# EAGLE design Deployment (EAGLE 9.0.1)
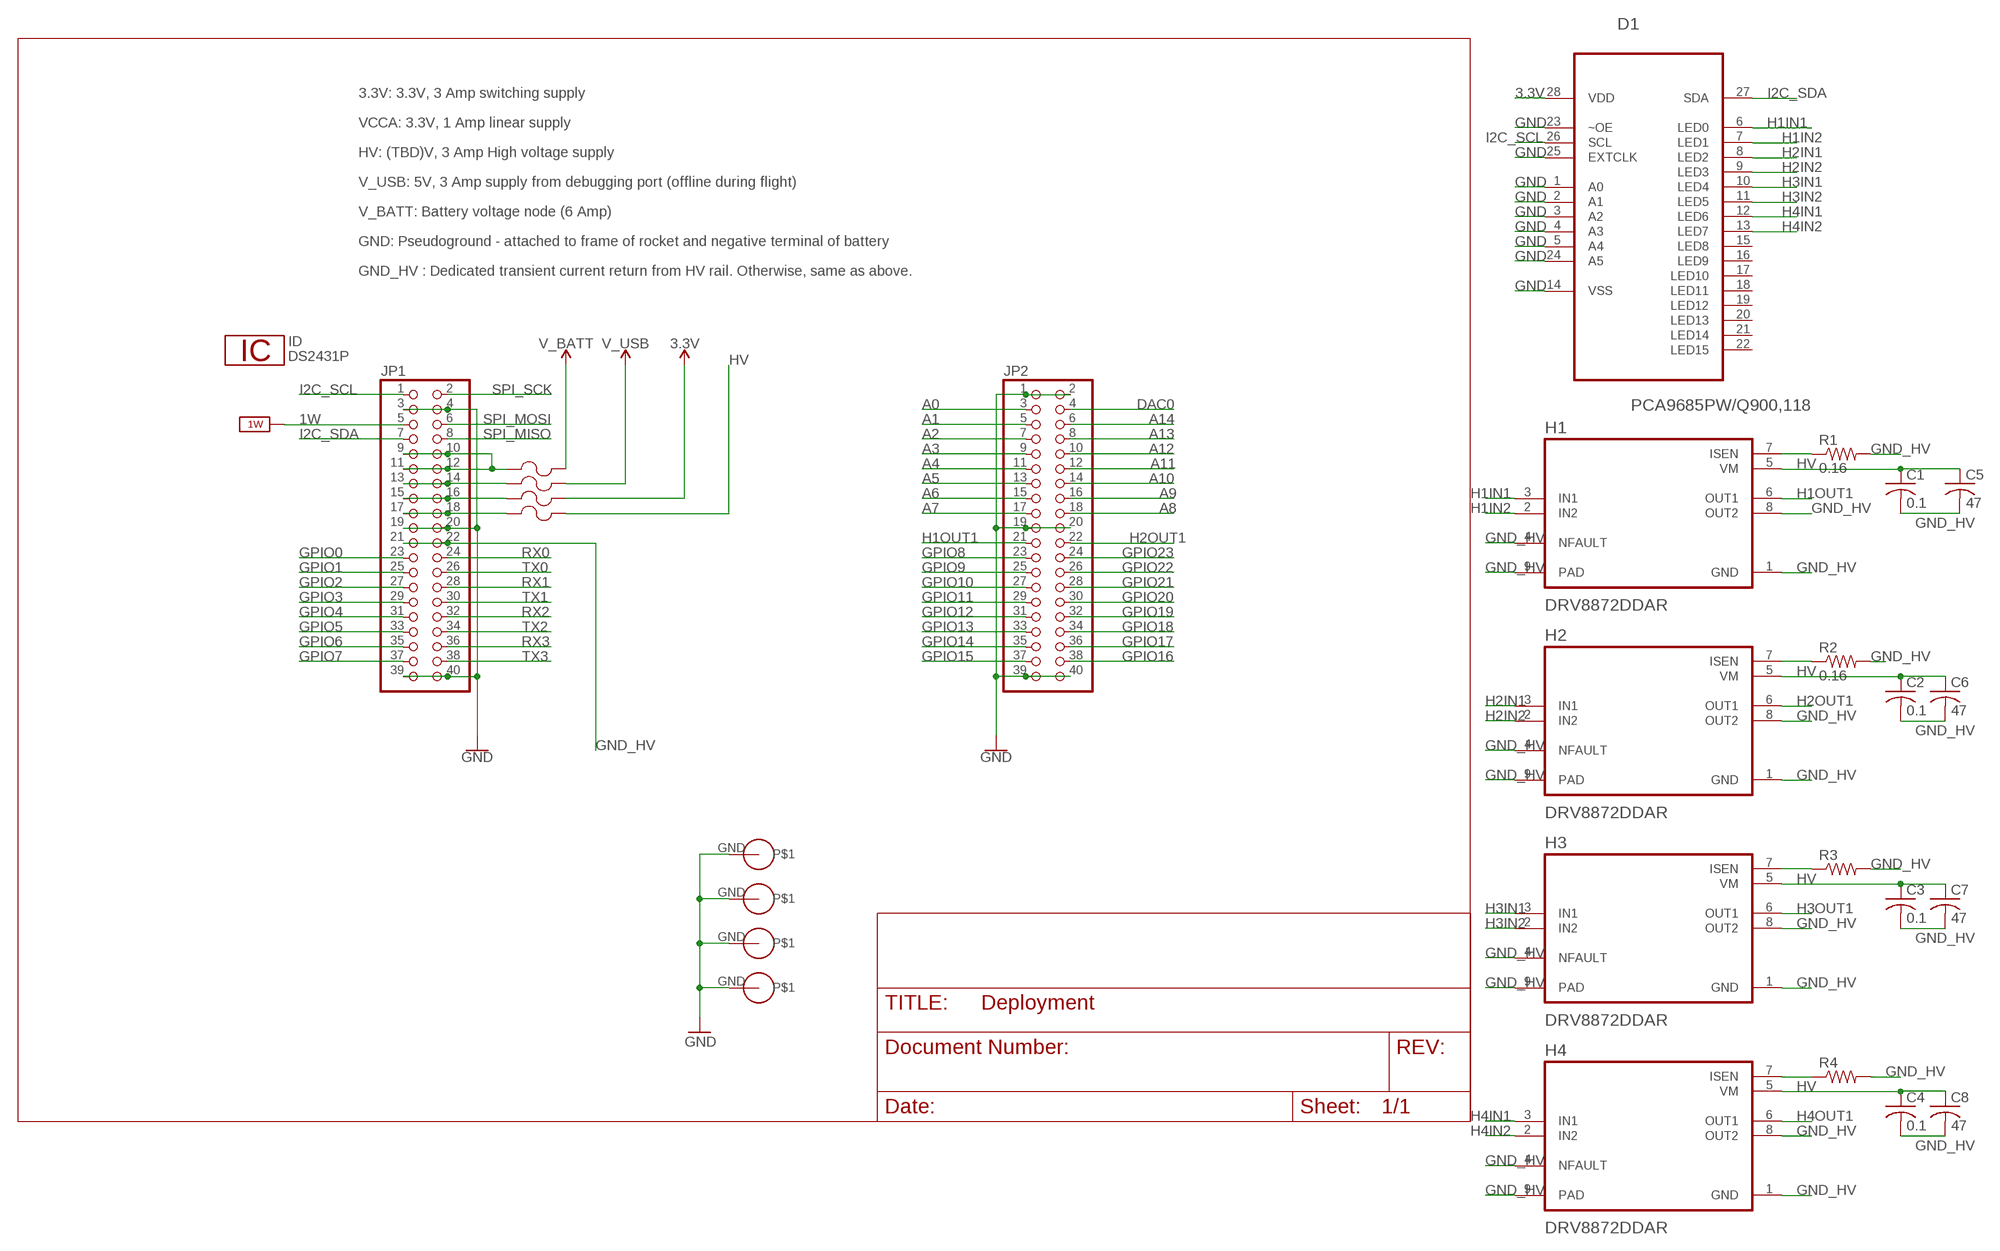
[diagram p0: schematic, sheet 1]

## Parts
C1  0.1  C-USC0805  [C0805]
C2  0.1  C-USC0805  [C0805]
C3  0.1  C-USC0805  [C0805]
C4  0.1  C-USC0805  [C0805]
C5  47  C-USC0805  [C0805]
C6  47  C-USC0805  [C0805]
C7  47  C-USC0805  [C0805]
C8  47  C-USC0805  [C0805]
D1  PCA9685PW/Q900,118  [SOP65P640X110-28N]
F1  0603SFF150F/32-2  [FUS0603_TYCO]
F2  0603SFF150F/32-2  [FUS0603_TYCO]
F3  0603SFF150F/32-2  [FUS0603_TYCO]
F4  0603SFF150F/32-2  [FUS0603_TYCO]
H1  DRV8872DDAR  [SOIC127P600X170-8N]
H2  DRV8872DDAR  [SOIC127P600X170-8N]
H3  DRV8872DDAR  [SOIC127P600X170-8N]
H4  DRV8872DDAR  [SOIC127P600X170-8N]
ID  DS2431P  [TSOC6]
JP1  PINHD-2X20  [2X20]
JP2  PINHD-2X20  [2X20]
R1  0.16  R-US_R1206  [R1206]
R2  0.16  R-US_R1206  [R1206]
R3  R-US_R1206  [R1206]
R4  R-US_R1206  [R1206]
U$1  PS/104-MOUNTING-HOLE  [PC/104-MOUNTING-HOLE]
U$2  PS/104-MOUNTING-HOLE  [PC/104-MOUNTING-HOLE]
U$3  PS/104-MOUNTING-HOLE  [PC/104-MOUNTING-HOLE]
U$4  PS/104-MOUNTING-HOLE  [PC/104-MOUNTING-HOLE]

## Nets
1W: JP1.5 ; supply symbol labelled 1W_SUP
3.3V: D1.28(VDD) F3.2
A0: JP2.3
A1: JP2.5
A2: JP2.7
A3: JP2.9
A4: JP2.11
A5: JP2.13
A6: JP2.15
A7: JP2.17
A8: JP2.18
A9: JP2.16
A10: JP2.14
A11: JP2.12
A12: JP2.10
A13: JP2.8
A14: JP2.6
DAC0: JP2.4
GND: D1.1(A0) D1.2(A1) D1.3(A2) D1.4(A3) D1.5(A4) D1.14(VSS) D1.23(~OE) D1.24(A5) D1.25(EXTCLK) JP1.3 JP1.4 JP1.19 JP1.20 JP1.39 JP1.40 JP2.1 JP2.2 JP2.19 JP2.20 JP2.39 JP2.40 U$1.GND U$2.GND U$3.GND U$4.GND
GND_HV: C1.2 C2.2 C3.2 C4.2 C5.2 C6.2 C7.2 C8.2 H1.1(GND) H1.4(NFAULT) H1.8(OUT2) H1.9(PAD) H2.1(GND) H2.4(NFAULT) H2.8(OUT2) H2.9(PAD) H3.1(GND) H3.4(NFAULT) H3.8(OUT2) H3.9(PAD) H4.1(GND) H4.4(NFAULT) H4.8(OUT2) H4.9(PAD) JP1.21 JP1.22 R1.2 R2.2 R3.2 R4.2
GPIO0: JP1.23
GPIO1: JP1.25
GPIO2: JP1.27
GPIO3: JP1.29
GPIO4: JP1.31
GPIO5: JP1.33
GPIO6: JP1.35
GPIO7: JP1.37
GPIO8: JP2.23
GPIO9: JP2.25
GPIO10: JP2.27
GPIO11: JP2.29
GPIO12: JP2.31
GPIO13: JP2.33
GPIO14: JP2.35
GPIO15: JP2.37
GPIO16: JP2.38
GPIO17: JP2.36
GPIO18: JP2.34
GPIO19: JP2.32
GPIO20: JP2.30
GPIO21: JP2.28
GPIO22: JP2.26
GPIO23: JP2.24
H1IN1: D1.6(LED0) H1.3(IN1)
H1IN2: D1.7(LED1) H1.2(IN2)
H1OUT1: H1.6(OUT1) JP2.21
H2IN1: D1.8(LED2) H2.3(IN1)
H2IN2: D1.9(LED3) H2.2(IN2)
H2OUT1: H2.6(OUT1) JP2.22
H3IN1: D1.10(LED4) H3.3(IN1)
H3IN2: D1.11(LED5) H3.2(IN2)
H3OUT1: H3.6(OUT1)
H4IN1: D1.12(LED6) H4.3(IN1)
H4IN2: D1.13(LED7) H4.2(IN2)
H4OUT1: H4.6(OUT1)
HV: C1.1 C2.1 C3.1 C4.1 C5.1 C6.1 C7.1 C8.1 F4.2 H1.5(VM) H2.5(VM) H3.5(VM) H4.5(VM)
I2C_SCL: D1.26(SCL) JP1.1
I2C_SDA: D1.27(SDA) JP1.7
N$1: F4.1 JP1.17 JP1.18
N$2: F2.1 JP1.13 JP1.14
N$3: F3.1 JP1.15 JP1.16
N$4: F1.1 JP1.9 JP1.10 JP1.11 JP1.12
N$5: H1.7(ISEN) R1.1
N$6: H2.7(ISEN) R2.1
N$10: H3.7(ISEN) R3.1
N$11: H4.7(ISEN) R4.1
RX0: JP1.24
RX1: JP1.28
RX2: JP1.32
RX3: JP1.36
SPI_MISO: JP1.8
SPI_MOSI: JP1.6
SPI_SCK: JP1.2
TX0: JP1.26
TX1: JP1.30
TX2: JP1.34
TX3: JP1.38
V_BATT: F1.2
V_USB: F2.2
Unconnected: D1.15(LED8) D1.16(LED9) D1.17(LED10) D1.18(LED11) D1.19(LED12) D1.20(LED13) D1.21(LED14) D1.22(LED15)

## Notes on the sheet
- 3.3V: 3.3V, 3 Amp switching supply
- VCCA: 3.3V, 1 Amp linear supply
- HV: (TBD)V, 3 Amp High voltage supply
- V_USB: 5V, 3 Amp supply from debugging port (offline during flight)
- V_BATT: Battery voltage node (6 Amp)
- GND: Pseudoground - attached to frame of rocket and negative terminal of battery
- GND_HV : Dedicated transient current return from HV rail. Otherwise, same as above.

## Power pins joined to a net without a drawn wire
1W: ID.2(1W)
GND: ID.1(GND)

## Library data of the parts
C1-C8 = resistor:C-US: CAPACITOR, American symbol
D1 = PCA9685PW_Q900_118:PCA9685PW/Q900,118: 16-channel, 12-bit PWM Fm+ I2C-bus LED controller; DESCRIPTION: PCA9685 Series 25 mA 5.5V 1 MHz 16-Ch 12-bit PWM Fm+ I2C-bus LED Controller; DIGI-KEY_PART_NUMBER: 568-5931-1-ND; DIGI-KEY_PURCHASE_URL: https://www.digikey.com/product-detail/en/nxp-usa-inc/PCA9685PW-Q900,118/568-5931-1-ND/2531218?utm_source=snapeda&utm_medium=aggregator&utm_campaign=symbol; MF: NXP USA; MP: PCA9685PW/Q900,118; PACKAGE: TSSOP-28 NXP Semiconductors
F1-F4 = CU inSpace 2019 Parts:0603SFF150F/32-2; MANUFACTURER_PART_NUMBER: 0603SFF150F322; VENDOR: Littelfuse Inc
H1-H4 = DRV8872DDAR:DRV8872DDAR: None; AVAILABILITY: Unavailable; DESCRIPTION: Brushed DC Motor Driver With PWM Control 6.5V to 45V 8-Pin SOPowerPAD T/R; MF: Texas Instruments; MP: DRV8872DDAR; PACKAGE: SO-8 Texas Instruments; PRICE: None
ID = 1wire:DS2431: 1024-Bit EEPROM
JP1 JP2 = pinhead:PINHD-2X20: PIN HEADER
R1-R4 = resistor:R-US_: RESISTOR, American symbol
U$1-U$4 = CU inSpace 2019 Parts:PS/104-MOUNTING-HOLE: Mounting hole for PC/104 board.

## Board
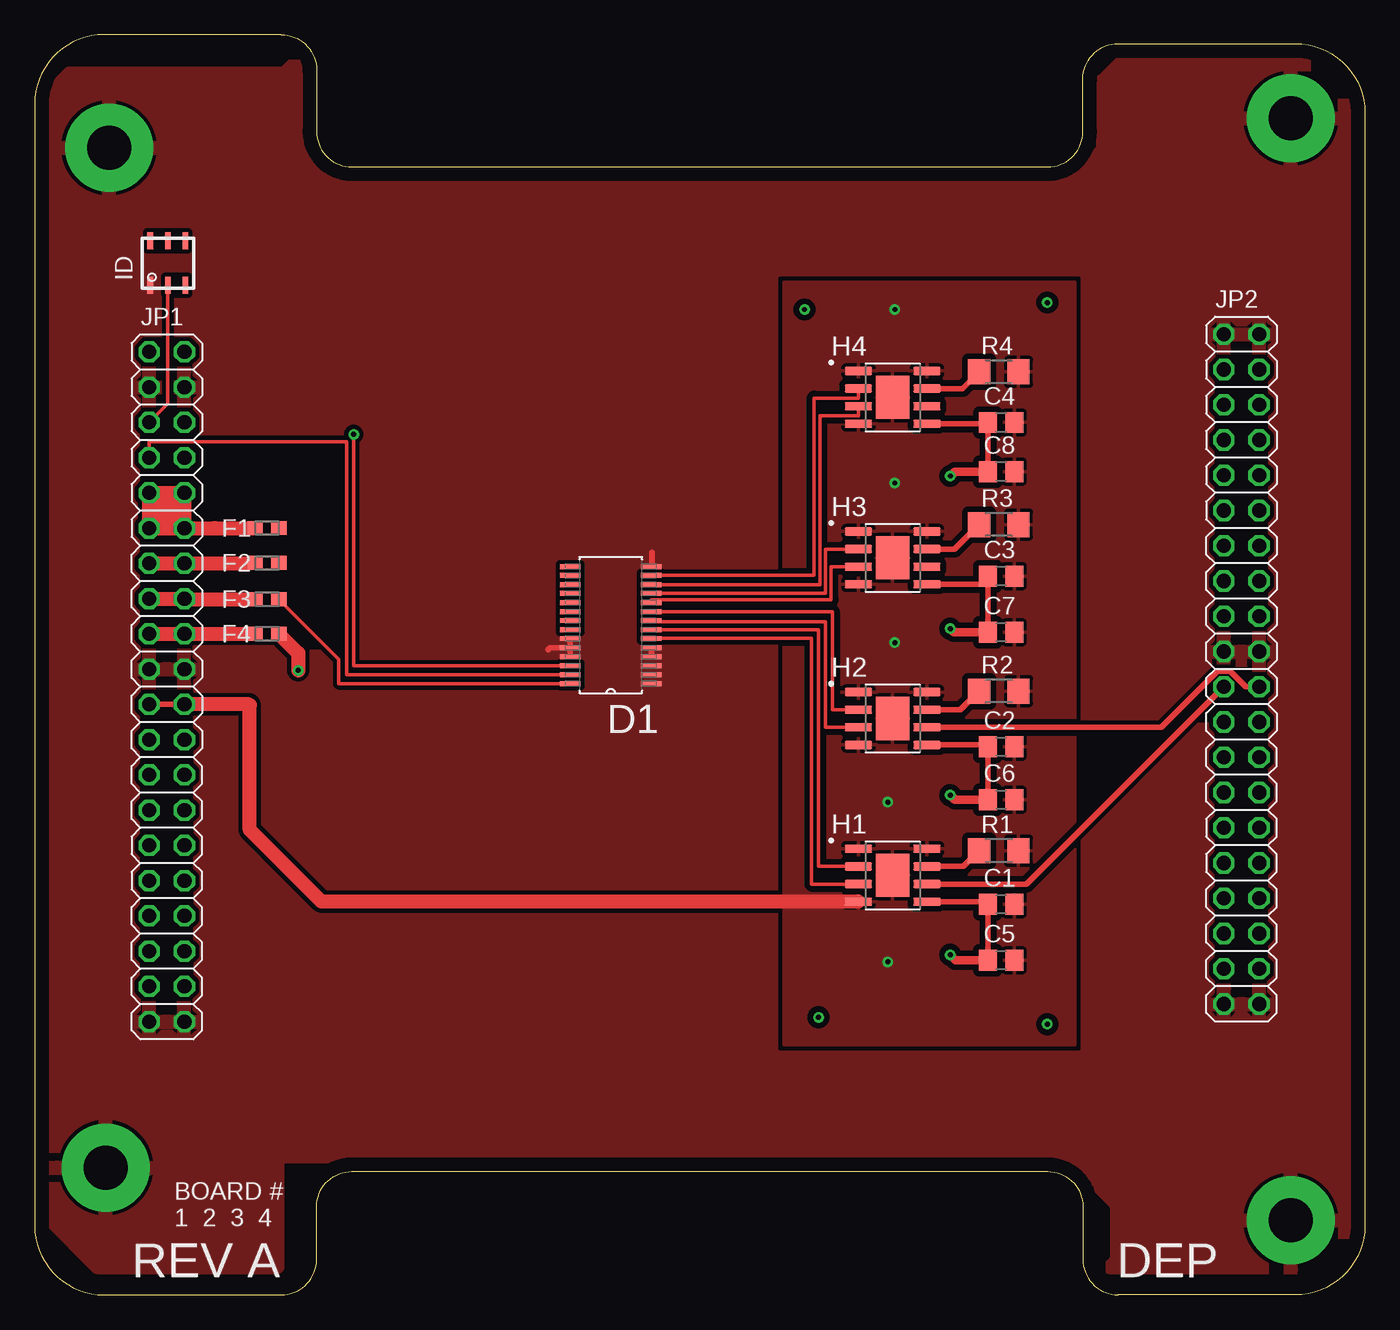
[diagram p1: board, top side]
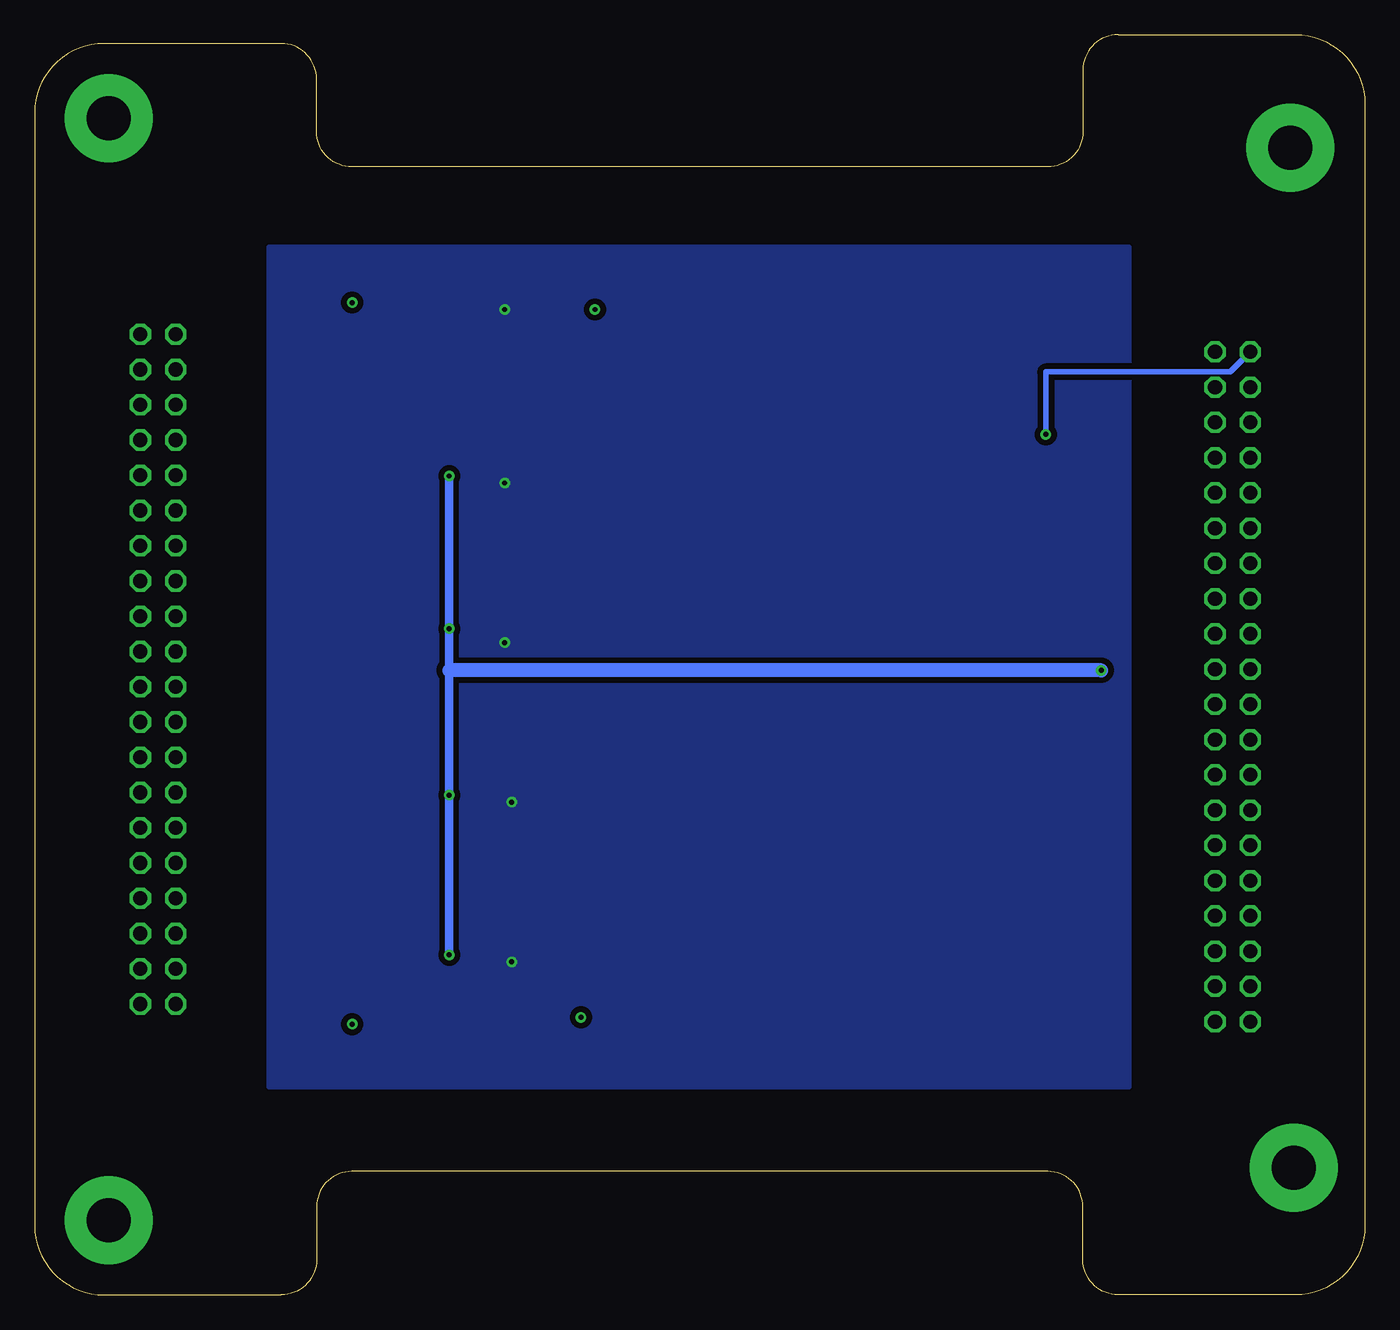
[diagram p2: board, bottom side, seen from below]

Size 95.89 x 90.81 mm. Coordinates in mm from the lower left corner, seen from the top.
Outline: 0,85.81 0,5 arc90 5,0 17.78,0 arc90 20.32,2.54 20.32,6.35 arc-90 22.86,8.89 73.03,8.89 arc-90 75.56,6.35 75.56,2.54 arc90 78.11,0 90.89,0 arc90 95.89,5 95.89,85.17 arc90 90.89,90.17 78.11,90.17 arc90 75.56,87.63 75.56,83.82 arc-90 73.03,81.28 22.86,81.28 arc-90 20.32,83.82 20.32,88.27 arc90 17.78,90.81 5,90.81 arc90 0,85.81
Copper layers (1*16): Top 0.035mm / dielectric 1.5mm / Bottom 0.035mm
Design rules "default": minimum track width 6mil, minimum drill 0.35mm, track to track 6mil, track to pad 6mil, pad to pad 6mil, via to via 6mil, smd to smd 6mil, copper to edge 40mil, drill to drill 6mil, minimum pad ring 10mil, minimum via ring 8mil, stop-mask expansion 4mil, vias tented up to drill 0mil, thermal gap 10mil

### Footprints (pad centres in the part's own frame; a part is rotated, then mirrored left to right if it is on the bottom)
C0805 = smd 1.3 x 1.5: 1 -0.95,0; 2 0.95,0
SOP65P640X110-28N = smd 1.473 x 0.356: 1 -2.921,4.216; 2 -2.921,3.581; 3 -2.921,2.921; 4 -2.921,2.286; 5 -2.921,1.626; 6 -2.921,0.965; 7 -2.921,0.33; 8 -2.921,-0.33; 9 -2.921,-0.965; 10 -2.921,-1.626; 11 -2.921,-2.286; 12 -2.921,-2.921; 13 -2.921,-3.581; 14 -2.921,-4.216; 15 2.921,-4.216; 16 2.921,-3.581; 17 2.921,-2.921; 18 2.921,-2.286; 19 2.921,-1.626; 20 2.921,-0.965; 21 2.921,-0.33; 22 2.921,0.33; 23 2.921,0.965; 24 2.921,1.626; 25 2.921,2.286; 26 2.921,2.921; 27 2.921,3.581; 28 2.921,4.216
FUS0603_TYCO = smd 1.092 x 0.991: 1 -0.851,0; 2 0.851,0
SOIC127P600X170-8N = smd 1.97 x 0.6: 1 -2.475,1.905; 2 -2.475,0.635; 3 -2.475,-0.635; 4 -2.475,-1.905; 5 2.475,-1.905; 6 2.475,-0.635; 7 2.475,0.635; 8 2.475,1.905 | smd 2.4 x 3.1: 9 0,0
TSOC6 = smd 0.406 x 1.219: 1 -1.27,-1.6; 2 0,-1.6; 3 1.27,-1.6; 4 1.27,1.6; 5 0,1.6; 6 -1.27,1.6
2X20 = drill 1.016 octagon: 1 -24.13,-1.27; 2 -24.13,1.27; 3 -21.59,-1.27; 4 -21.59,1.27; 5 -19.05,-1.27; 6 -19.05,1.27; 7 -16.51,-1.27; 8 -16.51,1.27; 9 -13.97,-1.27; 10 -13.97,1.27; 11 -11.43,-1.27; 12 -11.43,1.27; 13 -8.89,-1.27; 14 -8.89,1.27; 15 -6.35,-1.27; 16 -6.35,1.27; 17 -3.81,-1.27; 18 -3.81,1.27; 19 -1.27,-1.27; 20 -1.27,1.27; 21 1.27,-1.27; 22 1.27,1.27; 23 3.81,-1.27; 24 3.81,1.27; 25 6.35,-1.27; 26 6.35,1.27; 27 8.89,-1.27; 28 8.89,1.27; 29 11.43,-1.27; 30 11.43,1.27; 31 13.97,-1.27; 32 13.97,1.27; 33 16.51,-1.27; 34 16.51,1.27; 35 19.05,-1.27; 36 19.05,1.27; 37 21.59,-1.27; 38 21.59,1.27; 39 24.13,-1.27; 40 24.13,1.27
R1206 = smd 1.6 x 1.803: 1 -1.422,0; 2 1.422,0
PC/104-MOUNTING-HOLE = drill 3.175 pad 6.35: GND 0,0

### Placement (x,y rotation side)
C1  69.66,28.15 0 top
C2  69.66,39.5 0 top
C3  69.66,51.79 0 top
C4  69.66,62.86 0 top
C5  69.66,24.11 0 top
C6  69.66,35.68 0 top
C7  69.66,47.75 0 top
C8  69.66,59.32 0 top
D1  41.53,48.26 180 top
F1  16.75,55.25 0 top
F2  16.75,52.75 0 top
F3  16.75,50.13 0 top
F4  16.75,47.63 0 top
H1  61.85,30.23 0 top
H2  61.85,41.53 0 top
H3  61.85,53.1 0 top
H4  61.85,64.67 0 top
ID  9.6,74.35 0 top
JP1  9.53,43.81 270 top
JP2  87,45.09 270 top
R1  69.5,32 0 top
R2  69.5,43.5 0 top
R3  69.5,55.5 0 top
R4  69.5,66.5 0 top
U$1  5.36,82.65 0 top
U$2  90.55,84.79 0 top
U$3  5.13,9.17 0 top
U$4  90.55,5.36 0 top

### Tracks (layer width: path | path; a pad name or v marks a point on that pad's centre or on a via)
1W
  Top 0.254: ID.2 9.6,64.21 JP1.5
3.3V
  Top 0.254: D1.28 21.93,44.04 21.93,45.8 F3.2
GND
  Top 0.406: D1.24 37.13,46.63 37,46.5 | D1.25 D1.24 | D1.23 D1.24 | D1.5 D1.4 | D1.14 44.5,52.52 44.5,53.5
  pour Top (isolate 0.305, rank 2): 1,86 1,5.5 4.5,2 17.5,2 17.5,10 74.5,10 75,9.5 78,6.5 78,6 78,2.5 77.5,2 93.5,2 94.5,3 95,3 95,87 93,89 90.5,89 78.5,89 77,87.5 77,82.5 75,80.5 21,80.5 19,82.5 19,89 18,88 2.5,88 1,86.5
GND_HV  (via drill 0.35)
  Top 0.406: JP1.21 JP1.22
  Top 1.016: H1.4 20.68,28.32 15.5,33.5 15.5,42.5 15.46,42.55 JP1.22
  other vias: 62,71 62,58.5 62,47 61.5,35.5 61.5,24
  pour Top (isolate 0.406): 55,73 75,73 75,18 54,18 54,73
  pour Bottom (isolate 0.406): 17,75.5 79,75.5 79,15 17,15 17,75
H1IN1
  Top 0.254: D1.6 56,47.3 56,29.59 H1.3
H1IN2
  Top 0.254: D1.7 56.5,47.93 56.5,30.86 H1.2
H1OUT1
  Top 0.406: H1.6 71.5,29.59 JP2.21
H2IN1
  Top 0.254: D1.8 44.45,48.5 57,48.5 57,40.9 H2.3
H2IN2
  Top 0.254: D1.9 57.5,49.23 57.5,42.16 H2.2
H2OUT1
  Top 0.406: H2.6 81.22,40.9 85.26,44.93 86.19,44.93 87.31,43.81 JP2.22
H3IN1
  Top 0.254: D1.10 44.45,50.09 57.41,50.09 57.41,52.47 H3.3
H3IN2
  Top 0.254: D1.11 57,50.55 57,53.73 H3.2
H4IN1
  Top 0.254: D1.12 56.59,51.18 56.59,63.34 59.38,63.34 H4.3
H4IN2
  Top 0.254: D1.13 56.19,51.84 56.19,64.61 59.38,64.61 H4.2
HV  (via drill 0.35)
  Top 0.406: H2.5 68.58,39.62 C2.1 C6.1 | H3.5 68.11,51.2 C3.1 C7.1 | H1.5 68.53,28.32 C1.1 C5.1 | C8.1 C4.1 68.61,62.77 H4.5
  Top 0.61: C7.1 66.25,47.75 v66,48 | C6.1 66.32,35.68 v66,36 | C5.1 66.39,24.11 v66,24.5 | C8.1 66.32,59.32 v66,59
  Top 1.016: F4.2 19,46.24 v19,45
  Bottom 0.61: v66,59 v66,48 66,45 v66,36 v66,24.5
  Bottom 1.016: v19,45 66,45
I2C_SCL  (via drill 0.35)
  Top 0.254: D1.26 23,45.34 v23,62
  Bottom 0.406: JP1.1 9.7,66.5 10.31,66.5 10.33,66.52 11.26,66.52 11.28,66.5 23,66.5 v23,62
I2C_SDA
  Top 0.254: D1.27 22.5,44.68 22.5,61.47 8.26,61.47 JP1.7
N$1
  Top 1.016: JP1.17 JP1.18 14.9,47.62 F4.1
N$2
  Top 1.016: JP1.13 JP1.14 14.9,52.7 F2.1
N$3
  Top 1.016: JP1.15 JP1.16 10.79,50.13 F3.1
N$4
  Top 1.016: 9,55.24 JP1.11 JP1.9 | 9,55.24 10,55.24 | 10,55.24 JP1.12 | JP1.12 13,55.24 14.9,55.24 F1.1 | JP1.9 10,57.78 | 10,57.78 JP1.10 JP1.12 | JP1.9 9,57.78 9,55.24 | 10,55.24 10,57.78
N$5
  Top 0.406: R1.1 66.94,30.86 H1.7
N$6
  Top 0.406: R2.1 66.74,42.16 H2.7
N$7  (via drill 0.35)
  other vias: 56.5,20
N$8  (via drill 0.35)
  other vias: 73,19.5
N$9  (via drill 0.35)
  other vias: 55.5,71
N$10
  Top 0.406: R3.1 66.31,53.73 H3.7
N$11
  Top 0.406: R4.1 66.88,65.31 H4.7
N$12  (via drill 0.35)
  other vias: 73,71.5

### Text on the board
tPlace: BOARD # / 1 2 3 4 | REV A | DEP
Notes: RF Connectors should go in this notch | Debug connectors should go in this notch | Indicator LEDs should be placed in the bottom corners, filling the avaliable space from left to right

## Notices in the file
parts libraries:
SparkFun-PowerSymbols: Licensing: Creative Commons ShareAlike 4.0 International - https://creativecommons.org/licenses/by-sa/4.0
